| TEXAS INSTRUMENTS INCORPORATED
| Standard Linear and Logic Group
| IBIS Model of SN74LVC244A
| OCTAL BUFFER/DRIVER WITH 3-STATE OUTPUTS
| This file contains package information for the following:
|  TSSOP 20-pin (PW) package as [Component] LVC244J_PW
|  TVSOP 20-pin (DGV) package as [Component] LVC244J_DGV
|  SOIC 20-pin (DW) package as [Component] LVC244J_DW
|  SSOP 20-pin (DB) package as [Component] LVC244J_DB
|  QFN 20-pin (RGY) package as [Component] LVC244J_RGY
|  PDIP 20-pin (N) package as [Component] LVC244J_N
|  SOP 20-pin (NS) package as [Component] LVC244J_NS
|  jrBGA 20-pin (GQN) package as [Component] LVC244J_GQN
|  jrBGA 20-pin (ZQN) package as [Component] LVC244J_ZQN
| This device can be powered at the following Vccs:
|  1.8 volt Vcc
|  2.5 volt Vcc
|  3.3 volt Vcc
| This file provides unique models under the [Model Selector] for each Vcc.
| For operation at a specific Vcc, select the appropriate model after each
| [Model Selector] keyword.
[IBIS Ver]   3.2
[Comment char]  |_char
[File Name]   sn74lvc244a.ibs
[File Rev]   1.4 | j_die
[Date]   November 27, 2007
[Source]   Data created from TI-SPICE simulations at TI-SLL.
[Notes]   The following is an IBIS list for the SN74LVC244A.
   Please contact sllibis@ti.com with questions and
   comments concerning SLL IBIS models.
   - FILE REV HISTORY
   - 1.2 added RGY, DGV, N, and NS packages 01/29/04
   - 1.3 added GQN and ZQN packages 08/09/04
   - 1.4 recreated die data with updated simulation data 11/27/07
   - Power clamp data deleted as there is no power-clamp diode.
   - Though we took all possible cautions, there are some
   Ramp End points mismatch warnings in this file.
   - Due to the fact that the Device is 5-V Input/Output
   tolarent, the Model has some Non-Monotonic Warnings.
[Disclaimer] Property of Texas Instruments Incorporated.  Unauthorized
   reproduction and/or distribution is strictly prohibited.
   This product is protected under copyright law.
   Created  2007, (C) Copyright  2007, Texas Instruments
   Incorporated, All Rights Reserved
   UNLESS THERE IS A SIGNED, WRITTEN AGREEMENT TO THE
   CONTRARY, TEXAS INSTRUMENTS (TI) IS PROVIDING THE IBIS
   MODELS  AND WITHOUT ANY WARRANTY, EXPRESSED OR
   IMPLIED.  TI assumes no liability for:
   1) the accuracy of the IBIS models provided to your
   company;
   2) the proper functioning of these IBIS Models in your
   design or for any resulting applications; or
   3) infringement of patents, copyrights or intellectual
   property rights resulting from your use of these IBIS
   models.
   TI provides IBIS Models as a service to our customers.
   You and your company shall not distribute, sell or give
   these models to anyone else without prior written
   permission from TI.
   TI reserves the right to make changes to our products or
   to discontinue any semiconductor product or service
   without notice, and advises our customers to obtain the
   latest version of relevant information to verify, before
   placing orders, that the information being relied on is
   current.
   Please be aware that your receipt and use of the IBIS
   information provided shall serve as acceptance of these
   terms and conditions.  If you do not accept these terms,
   you should return or destroy the IBIS models and any
   other accompanying information immediately.
| Component SN74LVC244A_PW 20-PIN TSSOP
[Component]   SN74LVC244A_PW
[Manufacturer]   Texas Instruments, Inc.
[Package]
|   typ   min   max
R_pkg   5.000e-02   4.200e-02   6.000e-02
L_pkg   2.802e-09   2.248e-09   3.553e-09
C_pkg   3.170e-13   2.020e-13   4.430e-13
[Pin]   signal_name   model_name   R_pin   L_pin   C_pin
1   1NOE   LVC244A_NOE   5.500e-02   3.461e-09   4.400e-13
2   1A1   LVC244A_IN   5.500e-02   3.150e-09   4.010e-13
3   2Y4   LVC244A_OUT   4.200e-02   2.619e-09   3.020e-13
4   1A2   LVC244A_IN   4.500e-02   2.273e-09   2.020e-13
5   2Y3   LVC244A_OUT   4.500e-02   2.248e-09   2.240e-13
6   1A3   LVC244A_IN   4.500e-02   2.273e-09   2.260e-13
7   2Y2   LVC244A_OUT   4.400e-02   2.323e-09   2.050e-13
8   1A4   LVC244A_IN   4.600e-02   2.704e-09   3.070e-13
9   2Y1   LVC244A_OUT   6.000e-02   3.265e-09   4.110e-13
10   GND   GND   5.700e-02   3.506e-09   4.360e-13
11   2A1   LVC244A_IN   5.800e-02   3.553e-09   4.370e-13
12   1Y4   LVC244A_OUT   5.800e-02   3.193e-09   4.050e-13
13   2A2   LVC244A_IN   4.200e-02   2.704e-09   3.110e-13
14   1Y3   LVC244A_OUT   4.600e-02   2.392e-09   2.100e-13
15   2A3   LVC244A_IN   4.700e-02   2.334e-09   2.290e-13
16   1Y2   LVC244A_OUT   4.700e-02   2.300e-09   2.270e-13
17   2A4   LVC244A_IN   4.700e-02   2.349e-09   2.070e-13
18   1Y1   LVC244A_OUT   4.500e-02   2.677e-09   3.060e-13
19   2NOE   LVC244A_NOE   6.000e-02   3.235e-09   4.060e-13
20   VCC   POWER   5.600e-02   3.487e-09   4.430e-13
| Component SN74LVC244A_DGV 20-PIN TVSOP
[Component]   SN74LVC244A_DGV
[Manufacturer]   Texas Instruments, Inc.
[Package]
|   typ   min   max
R_pkg   4.400e-02   3.800e-02   4.800e-02
L_pkg   2.561e-09   2.236e-09   2.961e-09
C_pkg   3.420e-13   2.640e-13   4.460e-13
[Pin]   signal_name   model_name   R_pin   L_pin   C_pin
1   1NOE   LVC244A_NOE   4.400e-02   2.935e-09   4.170e-13
2   1A1   LVC244A_IN   4.200e-02   2.869e-09   4.460e-13
3   2Y4   LVC244A_OUT   4.300e-02   2.399e-09   3.160e-13
4   1A2   LVC244A_IN   4.400e-02   2.236e-09   2.650e-13
5   2Y3   LVC244A_OUT   4.600e-02   2.278e-09   2.640e-13
6   1A3   LVC244A_IN   4.500e-02   2.274e-09   2.640e-13
7   2Y2   LVC244A_OUT   4.400e-02   2.285e-09   2.690e-13
8   1A4   LVC244A_IN   4.300e-02   2.452e-09   3.200e-13
9   2Y1   LVC244A_OUT   4.400e-02   2.900e-09   4.460e-13
10   GND   GND   4.400e-02   2.961e-09   4.180e-13
11   2A1   LVC244A_IN   4.500e-02   2.954e-09   4.180e-13
12   1Y4   LVC244A_OUT   4.200e-02   2.847e-09   4.430e-13
13   2A2   LVC244A_IN   4.500e-02   2.453e-09   3.190e-13
14   1Y3   LVC244A_OUT   4.500e-02   2.297e-09   2.690e-13
15   2A3   LVC244A_IN   4.800e-02   2.334e-09   2.680e-13
16   1Y2   LVC244A_OUT   4.800e-02   2.335e-09   2.670e-13
17   2A4   LVC244A_IN   4.600e-02   2.299e-09   2.680e-13
18   1Y1   LVC244A_OUT   4.600e-02   2.457e-09   3.200e-13
19   2NOE   LVC244A_NOE   4.300e-02   2.848e-09   4.410e-13
20   VCC   POWER   3.800e-02   2.812e-09   4.080e-13
| Component SN74LVC244A_DW 20-PIN SOIC
[Component]   SN74LVC244A_DW
[Manufacturer]   Texas Instruments, Inc.
[Package]
|   typ   min   max
R_pkg   3.800e-02   3.300e-02   4.500e-02
L_pkg   5.012e-09   4.110e-09   6.349e-09
C_pkg   7.170e-13   5.300e-13   8.680e-13
[Pin]   signal_name   model_name   R_pin   L_pin   C_pin
1   1NOE   LVC244A_NOE   4.200e-02   6.336e-09   8.650e-13
2   1A1   LVC244A_IN   4.300e-02   5.542e-09   8.670e-13
3   2Y4   LVC244A_OUT   3.400e-02   4.714e-09   7.320e-13
4   1A2   LVC244A_IN   3.400e-02   4.377e-09   5.910e-13
5   2Y3   LVC244A_OUT   3.600e-02   4.130e-09   5.330e-13
6   1A3   LVC244A_IN   3.500e-02   4.111e-09   5.300e-13
7   2Y2   LVC244A_OUT   3.400e-02   4.284e-09   5.830e-13
8   1A4   LVC244A_IN   3.400e-02   4.634e-09   7.260e-13
9   2Y1   LVC244A_OUT   4.000e-02   5.518e-09   8.650e-13
10   GND   GND   4.300e-02   6.349e-09   8.660e-13
11   2A1   LVC244A_IN   4.100e-02   6.281e-09   8.610e-13
12   1Y4   LVC244A_OUT   4.500e-02   5.561e-09   8.680e-13
13   2A2   LVC244A_IN   3.300e-02   4.778e-09   7.420e-13
14   1Y3   LVC244A_OUT   3.500e-02   4.414e-09   5.960e-13
15   2A3   LVC244A_IN   3.500e-02   4.110e-09   5.330e-13
16   1Y2   LVC244A_OUT   3.600e-02   4.130e-09   5.330e-13
17   2A4   LVC244A_IN   3.400e-02   4.377e-09   5.910e-13
18   1Y1   LVC244A_OUT   3.400e-02   4.714e-09   7.310e-13
19   2NOE   LVC244A_NOE   4.300e-02   5.569e-09   8.680e-13
20   VCC   POWER   4.200e-02   6.308e-09   8.640e-13
| Component SN74LVC244A_DB 20-PIN SSOP
[Component]   SN74LVC244A_DB
[Manufacturer]   Texas Instruments, Inc.
[Package]
|   typ   min   max
R_pkg   4.000e-02   3.500e-02   5.100e-02
L_pkg   3.495e-09   3.035e-09   4.314e-09
C_pkg   4.200e-13   3.460e-13   5.020e-13
[Pin]   signal_name   model_name   R_pin   L_pin   C_pin
1   1NOE   LVC244A_NOE   4.900e-02   4.310e-09   5.020e-13
2   1A1   LVC244A_IN   4.800e-02   3.903e-09   4.870e-13
3   2Y4   LVC244A_OUT   3.500e-02   3.189e-09   3.960e-13
4   1A2   LVC244A_IN   3.500e-02   3.036e-09   3.470e-13
5   2Y3   LVC244A_OUT   3.500e-02   3.035e-09   3.670e-13
6   1A3   LVC244A_IN   3.500e-02   3.035e-09   3.670e-13
7   2Y2   LVC244A_OUT   3.500e-02   3.036e-09   3.470e-13
8   1A4   LVC244A_IN   3.500e-02   3.189e-09   3.970e-13
9   2Y1   LVC244A_OUT   4.700e-02   3.899e-09   4.880e-13
10   GND   GND   5.100e-02   4.314e-09   5.000e-13
11   2A1   LVC244A_IN   5.100e-02   4.314e-09   5.000e-13
12   1Y4   LVC244A_OUT   4.700e-02   3.899e-09   4.880e-13
13   2A2   LVC244A_IN   3.500e-02   3.189e-09   3.970e-13
14   1Y3   LVC244A_OUT   3.500e-02   3.036e-09   3.460e-13
15   2A3   LVC244A_IN   3.500e-02   3.035e-09   3.670e-13
16   1Y2   LVC244A_OUT   3.500e-02   3.035e-09   3.670e-13
17   2A4   LVC244A_IN   3.500e-02   3.036e-09   3.460e-13
18   1Y1   LVC244A_OUT   3.500e-02   3.189e-09   3.970e-13
19   2NOE   LVC244A_NOE   4.700e-02   3.899e-09   4.880e-13
20   VCC   POWER   5.100e-02   4.314e-09   5.020e-13
| Component SN74LVC244A_RGY 20-PIN QFN
[Component]   SN74LVC244A_RGY
[Manufacturer]   Texas Instruments, Inc.
[Package]
|   typ   min   max
R_pkg   5.000e-02   4.600e-02   5.500e-02
L_pkg   1.119e-09   1.025e-09   1.227e-09
C_pkg   3.520e-13   3.440e-13   3.630e-13
[Pin]   signal_name   model_name   R_pin   L_pin   C_pin
1   1NOE   LVC244A_NOE   5.200e-02   1.167e-09   3.600e-13
2   1A1   LVC244A_IN   4.700e-02   1.049e-09   3.440e-13
3   2Y4   LVC244A_OUT   4.700e-02   1.055e-09   3.450e-13
4   1A2   LVC244A_IN   5.000e-02   1.119e-09   3.500e-13
5   2Y3   LVC244A_OUT   5.500e-02   1.227e-09   3.600e-13
6   1A3   LVC244A_IN   5.200e-02   1.167e-09   3.550e-13
7   2Y2   LVC244A_OUT   4.900e-02   1.087e-09   3.480e-13
8   1A4   LVC244A_IN   4.700e-02   1.054e-09   3.460e-13
9   2Y1   LVC244A_OUT   4.900e-02   1.091e-09   3.490e-13
10   GND   GND   5.300e-02   1.184e-09   3.620e-13
11   2A1   LVC244A_IN   5.300e-02   1.181e-09   3.600e-13
12   1Y4   LVC244A_OUT   5.000e-02   1.108e-09   3.490e-13
13   2A2   LVC244A_IN   4.800e-02   1.075e-09   3.470e-13
14   1Y3   LVC244A_OUT   5.000e-02   1.107e-09   3.490e-13
15   2A3   LVC244A_IN   5.400e-02   1.200e-09   3.620e-13
16   1Y2   LVC244A_OUT   5.100e-02   1.141e-09   3.570e-13
17   2A4   LVC244A_IN   4.700e-02   1.043e-09   3.440e-13
18   1Y1   LVC244A_OUT   4.600e-02   1.025e-09   3.440e-13
19   2NOE   LVC244A_NOE   4.900e-02   1.090e-09   3.490e-13
20   VCC   POWER   5.400e-02   1.204e-09   3.630e-13
| Component SN74LVC244A_N 20-PIN PDIP
[Component]   SN74LVC244A_N
[Manufacturer]   Texas Instruments, Inc.
[Package]
|   typ   min   max
R_pkg   4.300e-02   3.800e-02   5.000e-02
L_pkg   7.384e-09   4.680e-09   1.032e-08
C_pkg   5.100e-13   2.310e-13   8.210e-13
[Pin]   signal_name   model_name   R_pin   L_pin   C_pin
1   1NOE   LVC244A_NOE   4.200e-02   9.427e-09   8.100e-13
2   1A1   LVC244A_IN   4.600e-02   8.544e-09   4.560e-13
3   2Y4   LVC244A_OUT   4.800e-02   7.163e-09   4.350e-13
4   1A2   LVC244A_IN   4.000e-02   4.825e-09   2.610e-13
5   2Y3   LVC244A_OUT   4.000e-02   5.284e-09   6.480e-13
6   1A3   LVC244A_IN   4.000e-02   4.686e-09   2.320e-13
7   2Y2   LVC244A_OUT   4.000e-02   6.359e-09   4.890e-13
8   1A4   LVC244A_IN   3.800e-02   7.982e-09   4.750e-13
9   2Y1   LVC244A_OUT   4.300e-02   9.403e-09   4.750e-13
10   GND   GND   5.000e-02   1.032e-08   8.050e-13
11   2A1   LVC244A_IN   5.000e-02   1.028e-08   8.100e-13
12   1Y4   LVC244A_OUT   4.300e-02   9.383e-09   4.770e-13
13   2A2   LVC244A_IN   3.800e-02   7.978e-09   4.760e-13
14   1Y3   LVC244A_OUT   4.000e-02   6.302e-09   4.920e-13
15   2A3   LVC244A_IN   4.000e-02   4.680e-09   2.310e-13
16   1Y2   LVC244A_OUT   4.000e-02   5.284e-09   6.480e-13
17   2A4   LVC244A_IN   4.000e-02   4.822e-09   2.610e-13
18   1Y1   LVC244A_OUT   4.700e-02   7.118e-09   4.390e-13
19   2NOE   LVC244A_NOE   4.600e-02   8.492e-09   4.610e-13
20   VCC   POWER   4.300e-02   9.348e-09   8.210e-13
| Component SN74LVC244A_NS 20-PIN SOP
[Component]   SN74LVC244A_NS
[Manufacturer]   Texas Instruments, Inc.
[Package]
|   typ   min   max
R_pkg   4.400e-02   2.900e-02   5.800e-02
L_pkg   3.666e-09   2.317e-09   5.115e-09
C_pkg   5.480e-13   3.160e-13   7.250e-13
[Pin]   signal_name   model_name   R_pin   L_pin   C_pin
1   1NOE   LVC244A_NOE   5.800e-02   5.115e-09   7.250e-13
2   1A1   LVC244A_IN   5.300e-02   4.591e-09   7.240e-13
3   2Y4   LVC244A_OUT   4.900e-02   3.754e-09   5.720e-13
4   1A2   LVC244A_IN   2.900e-02   2.549e-09   3.880e-13
5   2Y3   LVC244A_OUT   3.100e-02   2.317e-09   3.160e-13
6   1A3   LVC244A_IN   3.100e-02   2.317e-09   3.160e-13
7   2Y2   LVC244A_OUT   2.900e-02   2.556e-09   3.990e-13
8   1A4   LVC244A_IN   4.900e-02   3.754e-09   5.790e-13
9   2Y1   LVC244A_OUT   5.300e-02   4.591e-09   7.240e-13
10   GND   GND   5.800e-02   5.115e-09   7.250e-13
11   2A1   LVC244A_IN   5.800e-02   5.115e-09   7.250e-13
12   1Y4   LVC244A_OUT   5.300e-02   4.591e-09   7.240e-13
13   2A2   LVC244A_IN   4.900e-02   3.754e-09   5.790e-13
14   1Y3   LVC244A_OUT   2.900e-02   2.557e-09   3.990e-13
15   2A3   LVC244A_IN   3.100e-02   2.317e-09   3.160e-13
16   1Y2   LVC244A_OUT   3.100e-02   2.317e-09   3.160e-13
17   2A4   LVC244A_IN   2.900e-02   2.557e-09   3.990e-13
18   1Y1   LVC244A_OUT   4.900e-02   3.754e-09   5.790e-13
19   2NOE   LVC244A_NOE   5.300e-02   4.591e-09   7.240e-13
20   VCC   POWER   5.800e-02   5.115e-09   7.250e-13
| Component SN74LVC244A_GQN 20-PIN JRBGA
[Component]   SN74LVC244A_GQN
[Manufacturer]   Texas Instruments, Inc.
[Package]
|   typ   min   max
R_pkg   4.300e-02   3.300e-02   6.100e-02
L_pkg   1.317e-09   8.960e-10   2.088e-09
C_pkg   1.130e-13   6.400e-14   1.900e-13
[Pin]   signal_name   model_name   R_pin   L_pin   C_pin
A2   1NOE   LVC244A_NOE   3.800e-02   1.199e-09   1.210e-13
A1   1A1   LVC244A_IN   4.000e-02   1.067e-09   1.020e-13
B3   2Y4   LVC244A_OUT   6.100e-02   1.999e-09   1.900e-13
B1   1A2   LVC244A_IN   3.300e-02   9.630e-10   7.100e-14
C2   2Y3   LVC244A_OUT   4.900e-02   1.523e-09   1.230e-13
C1   1A3   LVC244A_IN   3.300e-02   8.960e-10   6.400e-14
D3   2Y2   LVC244A_OUT   6.100e-02   1.899e-09   1.640e-13
D1   1A4   LVC244A_IN   3.300e-02   8.980e-10   6.700e-14
E2   2Y1   LVC244A_OUT   4.900e-02   1.514e-09   1.280e-13
E1   GND   GND   3.600e-02   1.006e-09   9.400e-14
E3   2A1   LVC244A_IN   4.900e-02   1.683e-09   1.460e-13
E4   1Y4   LVC244A_OUT   3.300e-02   1.121e-09   8.900e-14
D2   2A2   LVC244A_IN   6.100e-02   2.088e-09   1.730e-13
D4   1Y3   LVC244A_OUT   3.300e-02   1.027e-09   7.100e-14
C3   2A3   LVC244A_IN   4.900e-02   1.558e-09   1.240e-13
C4   1Y2   LVC244A_OUT   3.300e-02   9.280e-10   6.700e-14
B2   2A4   LVC244A_IN   6.100e-02   1.921e-09   1.770e-13
B4   1Y1   LVC244A_OUT   3.300e-02   9.010e-10   7.700e-14
A4   2NOE   LVC244A_NOE   3.700e-02   9.900e-10   9.800e-14
A3   VCC   POWER   3.500e-02   1.168e-09   1.190e-13
| Component SN74LVC244A_ZQN 20-PIN JRBGA
[Component]   SN74LVC244A_ZQN
[Manufacturer]   Texas Instruments, Inc.
[Package]
|   typ   min   max
R_pkg   4.300e-02   3.300e-02   6.100e-02
L_pkg   1.317e-09   8.960e-10   2.088e-09
C_pkg   1.130e-13   6.400e-14   1.900e-13
[Pin]   signal_name   model_name   R_pin   L_pin   C_pin
A2   1NOE   LVC244A_NOE   3.800e-02   1.199e-09   1.210e-13
A1   1A1   LVC244A_IN   4.000e-02   1.067e-09   1.020e-13
B3   2Y4   LVC244A_OUT   6.100e-02   1.999e-09   1.900e-13
B1   1A2   LVC244A_IN   3.300e-02   9.630e-10   7.100e-14
C2   2Y3   LVC244A_OUT   4.900e-02   1.523e-09   1.230e-13
C1   1A3   LVC244A_IN   3.300e-02   8.960e-10   6.400e-14
D3   2Y2   LVC244A_OUT   6.100e-02   1.899e-09   1.640e-13
D1   1A4   LVC244A_IN   3.300e-02   8.980e-10   6.700e-14
E2   2Y1   LVC244A_OUT   4.900e-02   1.514e-09   1.280e-13
E1   GND   GND   3.600e-02   1.006e-09   9.400e-14
E3   2A1   LVC244A_IN   4.900e-02   1.683e-09   1.460e-13
E4   1Y4   LVC244A_OUT   3.300e-02   1.121e-09   8.900e-14
D2   2A2   LVC244A_IN   6.100e-02   2.088e-09   1.730e-13
D4   1Y3   LVC244A_OUT   3.300e-02   1.027e-09   7.100e-14
C3   2A3   LVC244A_IN   4.900e-02   1.558e-09   1.240e-13
C4   1Y2   LVC244A_OUT   3.300e-02   9.280e-10   6.700e-14
B2   2A4   LVC244A_IN   6.100e-02   1.921e-09   1.770e-13
B4   1Y1   LVC244A_OUT   3.300e-02   9.010e-10   7.700e-14
A4   2NOE   LVC244A_NOE   3.700e-02   9.900e-10   9.800e-14
A3   VCC   POWER   3.500e-02   1.168e-09   1.190e-13
| Model LVC244A_IN
[Model Selector]   LVC244A_IN
LVC244A_IN_18   1.8 volt Vcc
LVC244A_IN_25   2.5 volt Vcc
LVC244A_IN_33   3.3 volt Vcc
| Model LVC244A_NOE
[Model Selector]   LVC244A_NOE
LVC244A_NOE_18   1.8 volt Vcc
LVC244A_NOE_25   2.5 volt Vcc
LVC244A_NOE_33   3.3 volt Vcc
| Model LVC244A_OUT
[Model Selector]   LVC244A_OUT
LVC244A_OUT_18   1.8 volt Vcc
LVC244A_OUT_25   2.5 volt Vcc
LVC244A_OUT_33   3.3 volt Vcc
| Models and submodels in the file (9): LVC244A_IN_18 (Input), LVC244A_IN_25 (Input), LVC244A_IN_33 (Input), LVC244A_NOE_18 (Input), LVC244A_NOE_25 (Input), LVC244A_NOE_33 (Input), LVC244A_OUT_18 (3-state), LVC244A_OUT_25 (3-state), LVC244A_OUT_33 (3-state)
